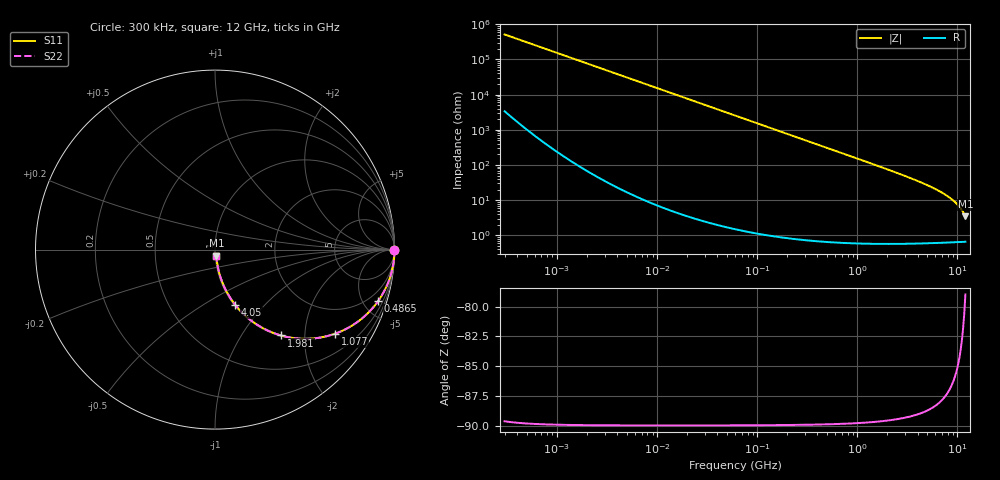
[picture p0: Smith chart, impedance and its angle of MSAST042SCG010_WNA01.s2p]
! MSAST042SCG010_WNA01  S-PARAMETER MODEL  ( General Type )
! Model Generated by TAIYO YUDEN Corporation (http://www.ty-top.com)
! Version 1.0
! TAIYO YUDEN Control No. 150820
! Copyright(c) 2015 TAIYO YUDEN CO.,LTD. All Rights Reserved.
! Product Description (link to TY-COMPAS)
! https://ds.yuden.co.jp/TYCOMPAS/or/detail?pn=MSAST042SCG010AWNA01&u=M
! Products Name : Multilayer Ceramic Capacitors
! Characteristics :
!  Capacitance : 1 pF , Rated Voltage : 25V , TCC : CG / C0G
!  Case Size : 0.4 x 0.2 / 0.016 x 0.008 [mm/inch] , Thickness : 0.2 / 0.008 [mm/inch]
!  (Conditions: Temperature = 25 degC , DC Bias Current/Voltage = 0A / 0V)
! External Node Assignments :
!  1  o---| |---o  2
! GND o---------o GND
! Frequency Range : 0.3MHz  -  12000MHz  [ 401 STEP ]
# MHz S RI R 50
! Freq[MHz].  S11 Real  S11 Imag  S21 Real  S21 Imag  S12 Real  S12 Imag  S22 Real  S22 Imag
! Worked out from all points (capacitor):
!   401 points, 300 kHz to 12 GHz, reference 50 ohm
!   read as one part in series: C = 1.03 pF near 316.3 kHz
!   lowest |Z| = 3.47 ohm at 12 GHz (marker M1)
!   S11 on the Smith chart (normalised r, x): 300 kHz: open; 486.5 MHz: 1.01, -6.32; 1.077 GHz: 1.01, -2.84; 1.981 GHz: 1.01, -1.52; 4.05 GHz: 1.01, -0.70; 12 GHz: 1.01, -0.07
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0.3  1 -0.000195  1.32e-06 0.000195  1.32e-06 0.000195  1 -0.000195
1.769972  1 -0.00115  2.42e-06 0.00115  2.42e-06 0.00115  1 -0.00115
10.44266  1 -0.00678  4.91e-05 0.00678  4.91e-05 0.00678  1 -0.00678
60  0.9985 -0.0389  0.00154 0.0389  0.00154 0.0389  0.9985 -0.0389
159.8975  0.9892 -0.1027  0.0108 0.1027  0.0108 0.1027  0.9892 -0.1027
237.9135  0.9765 -0.1509  0.0235 0.1509  0.0235 0.1509  0.9765 -0.1509
353.9943  0.9494 -0.2184  0.0506 0.2184  0.0506 0.2184  0.9494 -0.2184
486.4723  0.9085 -0.2872  0.0915 0.2872  0.0915 0.2872  0.9085 -0.2872
723.8279  0.8175 -0.3848  0.1825 0.3848  0.1825 0.3848  0.8175 -0.3848
1076.992  0.6681 -0.4688  0.3319 0.4688  0.3319 0.4688  0.6681 -0.4688
1480.043  0.514 -0.497  0.486 0.497  0.486 0.497  0.514 -0.497
1980.756  0.3681 -0.4785  0.6319 0.4785  0.6319 0.4785  0.3681 -0.4785
2088.533  0.3431 -0.4708  0.6569 0.4708  0.6569 0.4708  0.3431 -0.4708
2947.191  0.2023 -0.3959  0.7977 0.3959  0.7977 0.3959  0.2023 -0.3959
4050.141  0.1123 -0.3074  0.8877 0.3074  0.8877 0.3074  0.1123 -0.3074
6026.253  0.0469 -0.1972  0.9531 0.1972  0.9531 0.1972  0.0469 -0.1972
8064.993  0.022 -0.124  0.978 0.124  0.978 0.124  0.022 -0.124
8966.534  0.0163 -0.099  0.9837 0.099  0.9837 0.099  0.0163 -0.099
9968.853  0.0121 -0.0748  0.9879 0.0748  0.9879 0.0748  0.0121 -0.0748
10511.28  0.0105 -0.0629  0.9895 0.0629  0.9895 0.0629  0.0105 -0.0629
11380.75  0.0086 -0.0452  0.9914 0.0452  0.9914 0.0452  0.0086 -0.0452
12000  0.00772 -0.0336  0.9923 0.0336  0.9923 0.0336  0.00772 -0.0336
